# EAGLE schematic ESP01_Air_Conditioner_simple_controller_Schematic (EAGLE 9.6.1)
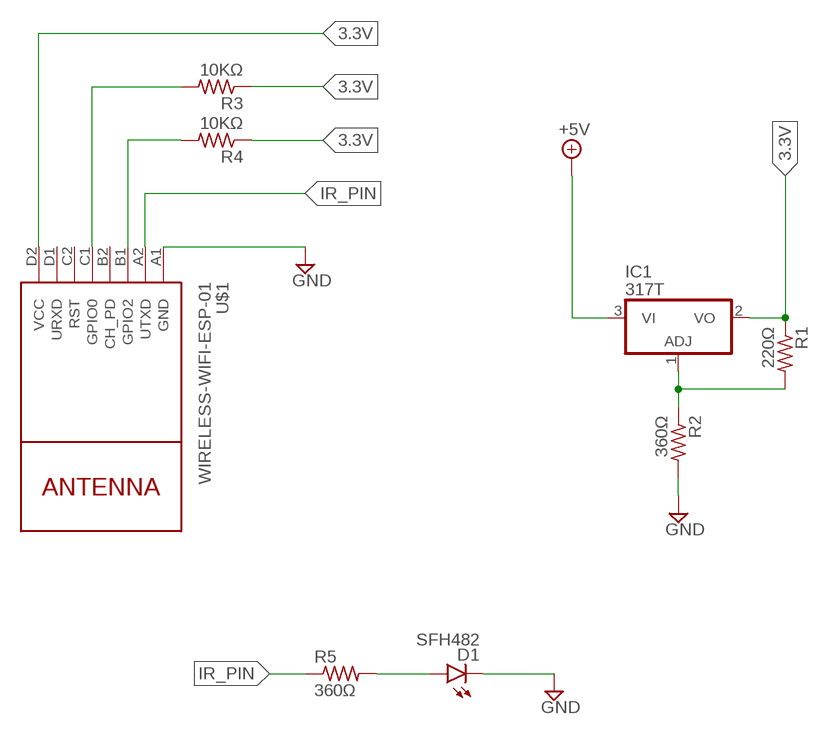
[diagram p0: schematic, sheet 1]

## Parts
D1  SFH482  [SFH482]
IC1  317T  [TO220H]
R1  220Ω  R-US_0204/5  [0204/5]
R2  360Ω  R-US_0204/5  [0204/5]
R3  10KΩ  R-US_0204/5  [0204/5]
R4  10KΩ  R-US_0204/5  [0204/5]
R5  360Ω  R-US_0204/5  [0204/5]
U$1  WIRELESS-WIFI-ESP-01  [WIRELESS-WIFI-ESP-01]

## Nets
3.3V: IC1.2(VO) R1.1 R3.1 R4.1 U$1.D2(VCC)
+5V: IC1.3(VI)
GND: D1.K(C) R2.2 U$1.A1(GND)
IR_PIN: U$1.A2(UTXD)
N$1: R4.2 U$1.B1(GPIO2)
N$2: IC1.1(ADJ) R1.2 R2.1
N$3: R3.2 U$1.C1(GPIO0)
N$4: R5.1
N$5: D1.A R5.2
Unconnected: U$1.B2(CH_PD) U$1.C2(RST) U$1.D1(URXD)

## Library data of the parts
D1 = led:SFH482: IR LED
IC1 = linear:*317: Positive VOLTAGE REGULATOR
R1-R5 = resistor:R-US_: RESISTOR, American symbol
U$1 = diy-modules:WIRELESS-WIFI-ESP-01: Wireless Wi-Fi ESP-01 Module based on ESP8266 chip Click here to find device on ebay.com

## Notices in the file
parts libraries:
diy-modules: Released under the Creative Commons Attribution 4.0 International License: http://creativecommons.org/licenses/by/4.0
